(* Logix 5000 AddOnInstructionDefinition export AMCI_3601_AOP_Configure; software revision 20.03 *)

ADD_ON_INSTRUCTION AMCI_3601_AOP_Configure   (* revision 0.0 *)
// Revision note:
// 3/2020: Version 0 is the initial release
// Help:
// The Limit Input can only be configured to have one function, ESTOP, CW Limit, or CCW Limit.  The 3401_Configure_AOI will disable the Limit Input if more than one type of functionality is selected.
VAR_INPUT
   Capture_Input : BOOL; {required}
   Capture_Input_Active_State : BOOL; {required}
   External_Input : BOOL; {required}
   External_Input_Active_State : BOOL; {required}
   Home_Input : BOOL; {required}
   Home_Input_Active_State : BOOL; {required}
   Emergency_Stop_Input : BOOL; {required}
   Emerency_Stop_Active_State : BOOL; {required}
   CW_Limit : BOOL; {required}
   CW_Limit_Active_State : BOOL; {required}
   CCW_Limit : BOOL; {required}
   CCW_Limit_Active_State : BOOL; {required}
   Backplane_Home_Proximity_Enable : BOOL;
   Quadrature_Encoder : BOOL; {required}
   Diagnostic_Feedback : BOOL;
   _0_for_CW_CCW_1_for_step_direction : BOOL; {required}
   _0_Home_Limit_1_Marker_Pulse_Home : BOOL;
   starting_speed : DINT; {required}
END_VAR
VAR_IN_OUT
   AMCI_3601_output_data : AM:1769_3601:O:0; {required}
END_VAR
VAR
   upper_result_X_1000 : DINT;
   command_data_block : INT[8];
        [0].15   // Mode Bit 1=Configuraiton Mode 0=Command Mode
END_VAR

ROUTINE Logic   (* ladder *)
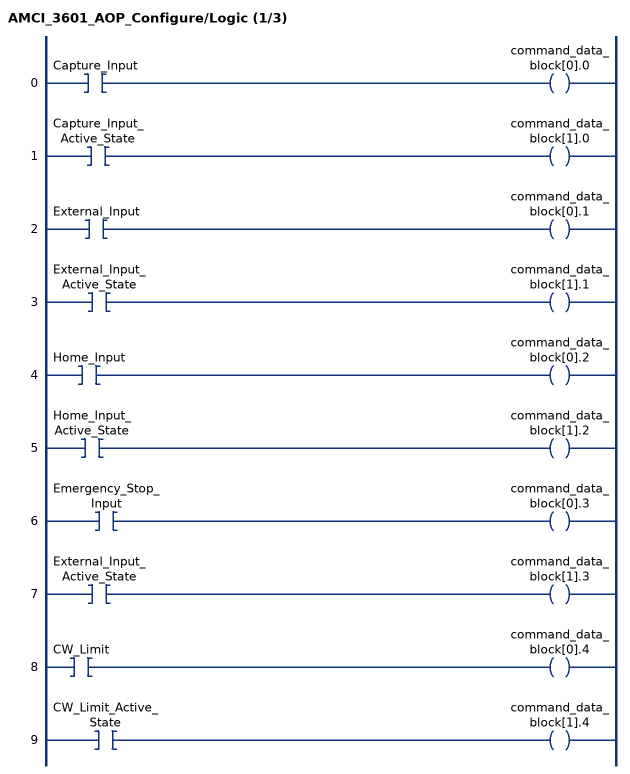
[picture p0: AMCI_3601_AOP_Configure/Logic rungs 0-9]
   0: XIC(Capture_Input)OTE(command_data_block[0].0);
   1: XIC(Capture_Input_Active_State)OTE(command_data_block[1].0);
   2: XIC(External_Input)OTE(command_data_block[0].1);
   3: XIC(External_Input_Active_State)OTE(command_data_block[1].1);
   4: XIC(Home_Input)OTE(command_data_block[0].2);
   5: XIC(Home_Input_Active_State)OTE(command_data_block[1].2);
   6: XIC(Emergency_Stop_Input)OTE(command_data_block[0].3);
   7: XIC(External_Input_Active_State)OTE(command_data_block[1].3);
   8: XIC(CW_Limit)OTE(command_data_block[0].4);
   9: XIC(CW_Limit_Active_State)OTE(command_data_block[1].4);
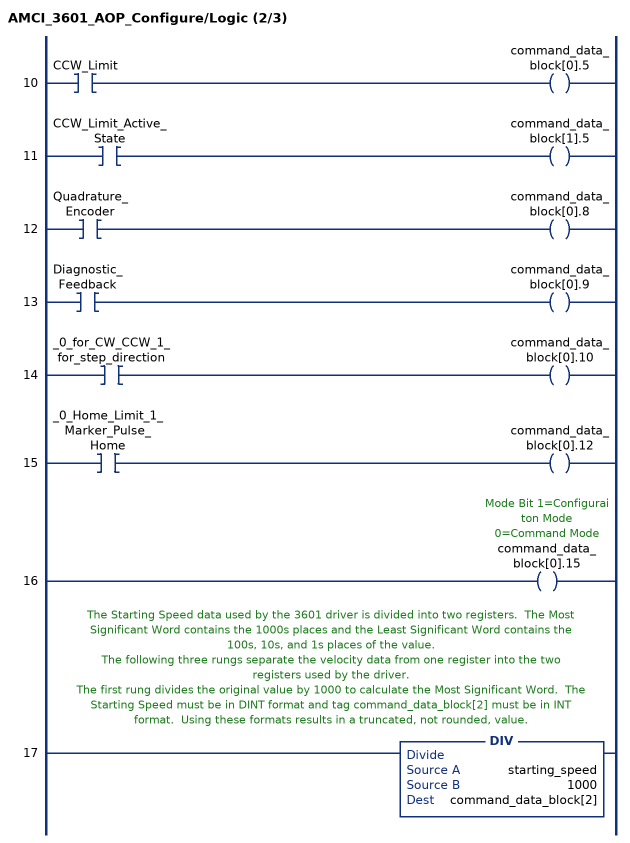
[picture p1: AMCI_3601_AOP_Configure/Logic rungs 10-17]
   10: XIC(CCW_Limit)OTE(command_data_block[0].5);
   11: XIC(CCW_Limit_Active_State)OTE(command_data_block[1].5);
   12: XIC(Quadrature_Encoder)OTE(command_data_block[0].8);
   13: XIC(Diagnostic_Feedback)OTE(command_data_block[0].9);
   14: XIC(_0_for_CW_CCW_1_for_step_direction)OTE(command_data_block[0].10);
   15: XIC(_0_Home_Limit_1_Marker_Pulse_Home)OTE(command_data_block[0].12);
   16: OTE(command_data_block[0].15);
   // The Starting Speed data used by the 3601 driver is divided into two registers.  The Most Significant Word contains the 1000s places and the Least Significant Word contains the 100s, 10s, and 1s places of the value.
   // The following three rungs separate the velocity data from one register into the two registers used by the driver.
   // The first rung divides the original value by 1000 to calculate the Most Significant Word.  The Starting Speed must be in DINT format and tag command_data_block[2] must be in INT format.  Using these formats results in a truncated, not rounded, value.
   17: DIV(starting_speed,1000,command_data_block[2]);
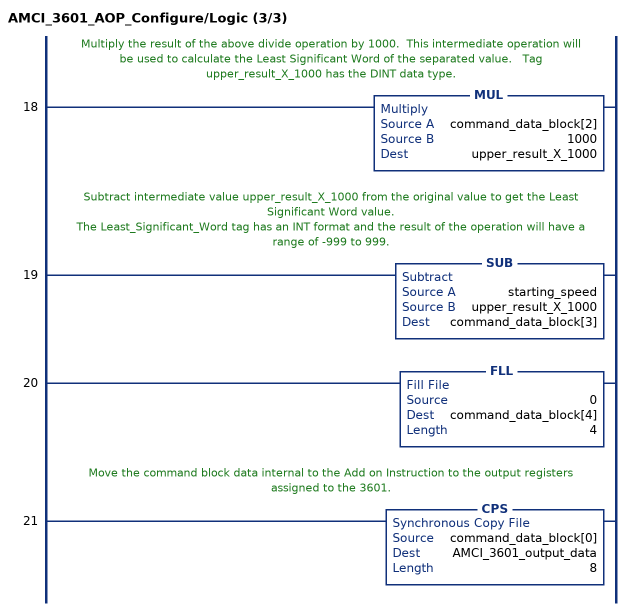
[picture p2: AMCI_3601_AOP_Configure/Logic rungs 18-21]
   // Multiply the result of the above divide operation by 1000.  This intermediate operation will be used to calculate the Least Significant Word of the separated value.   Tag upper_result_X_1000 has the DINT data type.
   18: MUL(command_data_block[2],1000,upper_result_X_1000);
   // Subtract intermediate value upper_result_X_1000 from the original value to get the Least Significant Word value.
   // The Least_Significant_Word tag has an INT format and the result of the operation will have a range of -999 to 999.
   19: SUB(starting_speed,upper_result_X_1000,command_data_block[3]);
   20: FLL(0,command_data_block[4],4);
   // Move the command block data internal to the Add on Instruction to the output registers assigned to the 3601.
   21: CPS(command_data_block[0],AMCI_3601_output_data,8);
END_ROUTINE
END_ADD_ON_INSTRUCTION
